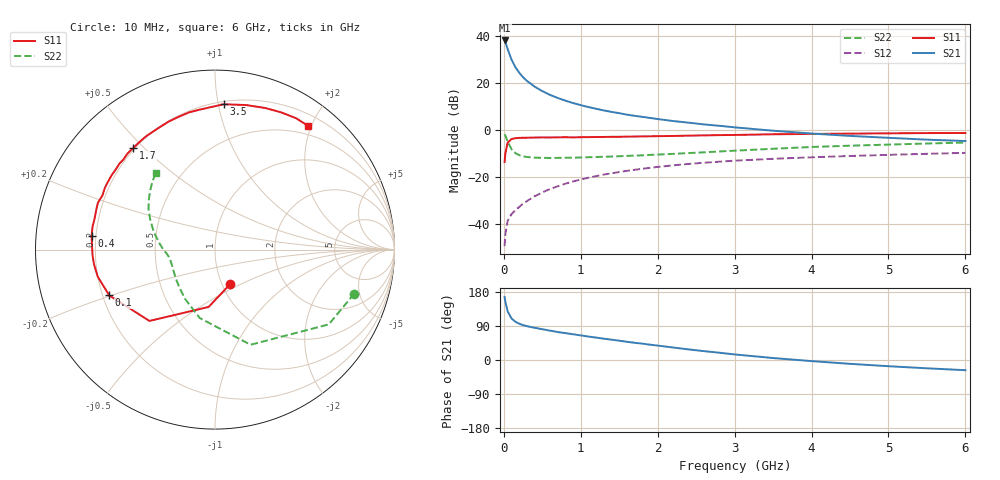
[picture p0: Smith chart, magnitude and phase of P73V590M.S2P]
! SIEMENS Small Signal Semiconductors
! BFP196
! Si NPN RF Bipolar Junction Transistor in SOT143
! VCE = 3.5 V  IC = 90 mA
! Common Emitter S-Parameters:  May  1996
# GHz  S  MA  R  50
!  f  S11  S21  S12  S22
! GHz  MAG  ANG  MAG  ANG  MAG  ANG  MAG  ANG
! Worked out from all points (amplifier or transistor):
!   36 points, 10 MHz to 6 GHz, reference 50 ohm
!   highest |S21| = 38.0 dB at 10 MHz (marker M1)
!   |S21| within 3 dB of that: start of sweep to 42.8 MHz
!   unconditionally stable (mu >= 1): 337.1 MHz to 4.644 GHz
!   at 250 MHz: K = 0.93, MSG = 26.9 dB, |S12| = -31.3 dB
!   at 1.4 GHz: K = 1.09, MAG = 11.2 dB, |S12| = -18.4 dB
!   at 6 GHz: K = 0.98, MSG = 2.5 dB, |S12| = -9.7 dB
!   S11 on the Smith chart (normalised r, x): 10 MHz: 1.10, -0.44; 100 MHz: 0.23, -0.20; 400 MHz: 0.18, +0.05; 1.7 GHz: 0.19, +0.46; 3.5 GHz: 0.22, +1.04; 6 GHz: 0.36, +1.96
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0.01  0.2091 -65.7  79.84 166.2  0.0034 76.2  0.8139 -17.5
0.02  0.3214 -96.3  73.02 153.1  0.0062 70.1  0.7588 -33.3
0.05  0.5399 -132.6  52.13 128.1  0.0118 54.2  0.566 -69.5
0.1  0.6421 -156.6  31.09 109.6  0.0163 51.6  0.3906 -102.6
0.15  0.6705 -167.0  21.62 101.0  0.0198 54.4  0.3224 -120.8
0.2  0.679 -173.0  16.46 95.7  0.0232 57.7  0.2915 -132.4
0.25  0.6831 -177.3  13.19 92.0  0.0272 60.2  0.2753 -140.9
0.3  0.6844 179.3  11.05 89.3  0.0308 62.7  0.2672 -146.3
0.4  0.6917 173.8  8.355 85.0  0.0391 64.9  0.2582 -154.4
0.5  0.6942 169.4  6.687 81.2  0.047 66.3  0.2554 -159.5
0.6  0.6926 165.7  5.575 77.5  0.0557 66.1  0.2547 -163.0
0.7  0.6978 161.5  4.793 73.8  0.0637 65.9  0.2552 -165.6
0.9  0.6959 154.3  3.733 67.9  0.0807 64.2  0.2579 -169.6
1.1  0.7058 147.8  3.068 61.9  0.0967 62.1  0.2639 -172.5
1.3  0.711 141.0  2.604 56.2  0.113 59.1  0.2696 -175.1
1.7  0.7264 128.9  1.999 45.4  0.1426 53.6  0.2855 179.9
2.2  0.7463 115.4  1.551 33.0  0.1771 45.7  0.3105 173.8
2.8  0.7783 100.6  1.228 19.2  0.212 36.6  0.3499 164.9
3.5  0.8113 86.6  0.965 5.2  0.2443 26.4  0.399 154.9
4.5  0.8372 70.4  0.748 -10.1  0.2806 14.3  0.4637 142.6
5.5  0.8599 58.4  0.623 -21.9  0.3119 3.4  0.5161 132.4
6  0.863 52.9  0.583 -26.9  0.3266 -2.2  0.5403 127.5
